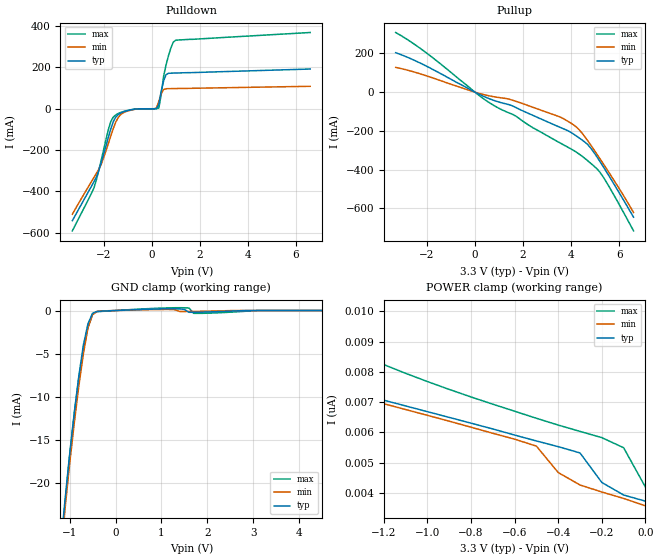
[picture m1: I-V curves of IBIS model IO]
|   TEXAS INSTRUMENTS INCORPORATED
|   Standard Linear and Logic
|   IBIS Model of SN74LVTH646
|   3.3V Octal Bus Transceiver Register (3-state)
|   24-pin DB, DGV, DW, or PW Package
[IBIS Ver]   2.1
[File Name]   lvth646.ibs
[File Rev]   1.0
[Date]   10/09/97
[Source]   File originated at Texas Instruments, Inc.
[Notes]   The following is an IBIS list for the LVTH646.
|   - This file may be incomplete or may not be fully compliant
|   with the IBIS specification. It will be replaced with a
|   version that is IBIS Revision 3.2 compliant and is complete
|   and accurate.  Please email all questions and comments to
|   sllibis@ti.com.
|   - All test data contained in this file are derived from
|   hspice(tm) simulations.
|   - File created by David Yaeger, SLL applications.
[Disclaimer]
* Property of Texas Instruments Incorporated.  Unauthorized *
* reproduction and/or distribution is strictly prohibited. *
* This product is protected under copyright law. *
* Created 1997, (C) Copyright 1997, Texas Instruments Inc., *
* All Rights Reserved *
* UNLESS THERE IS A SIGNED, WRITTEN AGREEMENT TO THE *
* CONTRARY, TEXAS INSTRUMENTS ("TI") IS PROVIDING THE IBIS *
* MODELS "AS IS" AND WITHOUT ANY WARRANTY, EXPRESSED OR *
* IMPLIED.  TI assumes no liability for: *
* 1) the accuracy of the IBIS models provided to your *
* company; *
* 2) the proper functioning of these IBIS models in your *
* design or for any resulting applications; or *
* 3) infringement of patents, copyrights or intellectual *
* property rights resulting from your use of these *
* IBIS models. *
* TI provides IBIS Models as a service to our customers. *
* You and your company shall not distribute, sell or give *
* these models to anyone else without prior written *
* permission from TI. *
* TI reserves the right to make changes to our products or *
* to discontinue any semiconductor product or service *
* without notice, and advises our customers to obtain the *
* latest version of relevant information to verify, before *
* placing orders, that the information being relied on is *
* current. *
* Please be aware that your receipt and use of the IBIS *
* information provided shall serve as acceptance of these *
* terms and conditions.  If you do not accept these terms, *
* you should return or destroy the IBIS models and any *
* other accompanying information immediately. *
[Component]   LVTH646_DB
[Manufacturer]  Texas Instruments, Inc.
[Package]
|   typ   min   max
R_pkg   0.045   0.04   0.049
L_pkg   3.668nH   3.226nH   4.415nH
C_pkg   0.416pF   0.349pF   0.507pF
[Pin]   signal_name   model_name   R_pin   L_pin   C_pin
1   CLKAB   NC   0.042   4.299nH   0.503pF
2   SAB   NC   0.04   3.96nH   0.499pF
3   DIR   NC   0.042   3.775nH   0.417pF
4   A1   IO   0.047   3.487nH   0.369pF
5   A2   IO   0.046   3.347nH   0.352pF
6   A3   IO   0.049   3.352nH   0.371pF
7   A4   IO   0.046   3.226nH   0.363pF
8   A5   IO   0.047   3.289nH   0.349pF
9   A6   IO   0.047   3.347nH   0.361pF
10   A7   IO   0.041   3.576nH   0.409pF
11   A8   IO   0.041   3.995nH   0.503pF
12   GND   GND   0.045   4.415nH   0.507pF
13   B8   IO   0.043   4.337nH   0.506pF
14   B7   IO   0.042   4.003nH   0.504pF
15   B6   IO   0.041   3.686nH   0.41pF
16   B5   IO   0.048   3.355nH   0.349pF
17   B4   IO   0.047   3.301nH   0.353pF
18   B3   IO   0.048   3.268nH   0.366pF
19   B2   IO   0.048   3.269nH   0.366pF
20   B1   IO   0.047   3.314nH   0.349pF
21   OE_BAR   NC   0.048   3.399nH   0.355pF
22   SBA   NC   0.041   3.688nH   0.412pF
23   CLKBA   NC   0.042   4.003nH   0.504pF
24   VCC   POWER   0.043   4.347nH   0.505pF
[Component]   LVTH646_DGV
[Manufacturer]  Texas Instruments, Inc.
[Package]
|   typ   min   max
R_pkg   0.043   0.039   0.047
L_pkg   2.601nH   2.312nH   3.626nH
C_pkg   0.358pF   0.277pF   0.595pF
[Pin]   signal_name   model_name   R_pin   L_pin   C_pin
1   CLKAB   NC   0.043   3.625nH   0.595pF
2   SAB   NC   0.04   2.656nH   0.402pF
3   DIR   NC   0.039   2.338nH   0.308pF
4   A1   IO   0.046   2.354nH   0.277pF
5   A2   IO   0.045   2.312nH   0.285pF
6   A3   IO   0.047   2.318nH   0.282pF
7   A4   IO   0.047   2.318nH   0.282pF
8   A5   IO   0.045   2.312nH   0.285pF
9   A6   IO   0.046   2.353nH   0.278pF
10   A7   IO   0.039   2.338nH   0.308pF
11   A8   IO   0.041   2.66nH   0.402pF
12   GND   GND   0.043   3.625nH   0.595pF
13   B8   IO   0.044   3.626nH   0.594pF
14   B7   IO   0.04   2.658nH   0.402pF
15   B6   IO   0.039   2.343nH   0.311pF
16   B5   IO   0.046   2.353nH   0.278pF
17   B4   IO   0.045   2.312nH   0.285pF
18   B3   IO   0.047   2.319nH   0.282pF
19   B2   IO   0.047   2.319nH   0.282pF
20   B1   IO   0.045   2.312nH   0.285pF
21   OE_BAR   NC   0.046   2.353nH   0.278pF
22   SBA   NC   0.039   2.337nH   0.308pF
23   CLKBA   NC   0.04   2.658nH   0.402pF
24   VCC   POWER   0.044   3.626nH   0.595pF
[Component]   LVTH646_DW
[Manufacturer]  Texas Instruments, Inc.
[Package]
|   typ   min   max
R_pkg   0.037   0.03   0.047
L_pkg   5.146nH   3.993nH   6.885nH
C_pkg   0.758pF   0.512pF   1.067pF
[Pin]   signal_name   model_name   R_pin   L_pin   C_pin
1   CLKAB   NC   0.039   6.885nH   1.067pF
2   SAB   NC   0.042   5.95nH   0.958pF
3   DIR   NC   0.047   5.317nH   0.791pF
4   A1   IO   0.031   4.651nH   0.611pF
5   A2   IO   0.03   3.993nH   0.512pF
6   A3   IO   0.03   4.083nH   0.611pF
7   A4   IO   0.03   4.083nH   0.611pF
8   A5   IO   0.03   3.993nH   0.512pF
9   A6   IO   0.031   4.652nH   0.611pF
10   A7   IO   0.047   5.317nH   0.791pF
11   A8   IO   0.042   5.95nH   0.959pF
12   GND   GND   0.039   6.885nH   1.067pF
13   B8   IO   0.039   6.885nH   1.067pF
14   B7   IO   0.042   5.95nH   0.959pF
15   B6   IO   0.047   5.317nH   0.791pF
16   B5   IO   0.031   4.652nH   0.611pF
17   B4   IO   0.03   3.993nH   0.512pF
18   B3   IO   0.03   4.083nH   0.61pF
19   B2   IO   0.03   4.083nH   0.61pF
20   B1   IO   0.03   3.993nH   0.512pF
21   OE_BAR   NC   0.031   4.651nH   0.611pF
22   SBA   NC   0.047   5.317nH   0.791pF
23   CLKBA   NC   0.042   5.95nH   0.958pF
24   VCC   POWER   0.039   6.885nH   1.067pF
[Component]   LVTH646_PW
[Manufacturer]  Texas Instruments, Inc.
[Package]
|   typ   min   max
R_pkg   0.039   0.03   0.046
L_pkg   2.685nH   2.367nH   3.177nH
C_pkg   0.32pF   0.252pF   0.434pF
[Pin]   signal_name   model_name   R_pin   L_pin   C_pin
1   CLKAB   NC   0.037   3.153nH   0.434pF
2   SAB   NC   0.034   2.629nH   0.341pF
3   DIR   NC   0.032   2.86nH   0.347pF
4   A1   IO   0.042   2.741nH   0.29pF
5   A2   IO   0.046   2.6nH   0.262pF
6   A3   IO   0.043   2.414nH   0.266pF
7   A4   IO   0.042   2.367nH   0.262pF
8   A5   IO   0.044   2.461nH   0.252pF
9   A6   IO   0.042   2.543nH   0.274pF
10   A7   IO   0.03   2.616nH   0.332pF
11   A8   IO   0.037   2.67nH   0.346pF
12   GND   GND   0.039   3.177nH   0.433pF
13   B8   IO   0.037   3.111nH   0.431pF
14   B7   IO   0.037   2.656nH   0.345pF
15   B6   IO   0.031   2.739nH   0.34pF
16   B5   IO   0.042   2.649nH   0.282pF
17   B4   IO   0.046   2.532nH   0.257pF
18   B3   IO   0.044   2.425nH   0.266pF
19   B2   IO   0.044   2.425nH   0.266pF
20   B1   IO   0.046   2.532nH   0.257pF
21   OE_BAR   NC   0.042   2.648nH   0.282pF
22   SBA   NC   0.031   2.738nH   0.339pF
23   CLKBA   NC   0.036   2.653nH   0.344pF
24   VCC   POWER   0.037   3.11nH   0.431pF
| Models and submodels in the file (1): IO (I/O)
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|   Model LVTH646_IO
[Model]   IO
Model_type   I/O
Polarity   Inverting
Enable   Active-Low
Vinl = 0.8V
Vinh = 2.0V
|   typ   min   max
C_comp   9pF   NA   NA
[Temperature Range]   50   0   100
[Voltage range]   3.3   3.0   3.6
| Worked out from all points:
|   slope of the pulldown table from 0 to 0.495 V, typ, clamps not added: 3.73 ohm
|   slope of the pullup table from 0 to 0.495 V, typ, clamps not added: 17.2 ohm
|   GND clamp passes 1 mA (typ) near -0.56 V on its own axis
[Pullup]   | Vtable = Vcc - Voutput
|   Voltage   I(typ)   I(min)   I(max)
-3.3V     203.6mA    127.8mA    307.8mA
-2V       132.9mA    83.47mA    200.5mA
500mV     -28.97mA   -16.47mA   -46.28mA
1.6V      -72.91mA   -43.01mA   -116.4mA
2.3V      -113.5mA   -72.99mA   -175.2mA
3.5V      -179.1mA   -126.1mA   -259mA
3.9V      -201.2mA   -152.7mA   -286.3mA
4.3V      -232.8mA   -189mA     -316.3mA
4.7V      -271.4mA   -251.8mA   -354.6mA
5.2V      -357.3mA   -342.7mA   -412.8mA
5.7V      -456.7mA   -438.2mA   -512.8mA
6.6V      -644.8mA   -620.7mA   -715.4mA
[Pulldown]
|   Voltage   I(typ)   I(min)   I(max)
-3.3V     -541.1mA   -510mA     -590.2mA
-2.4V     -352.7mA   -331.9mA   -382.4mA
-2.1V     -260.9mA   -270.2mA   -249.8mA
-1.8V     -138mA     -167.8mA   -100.2mA
-1.5V     -41.84mA   -66.63mA   -30.62mA
-1.2V     -16.44mA   -21.07mA   -14.61mA
200mV     117.8uA    3.002mA    -393.7uA
300mV     19.97mA    35.86mA    3.638mA
500mV     134.6mA    92.85mA    157.4mA
600mV     164.2mA    96.34mA    211.3mA
900mV     171.9mA    97.14mA    321.3mA
6.6V      191.6mA    108.1mA    368mA
[POWER_Clamp]   | Vtable = Vcc - Voutput
|   Voltage   I(typ)   I(min)   I(max)
-3.3V     11.05nA    10.98nA    33.46nA
-2.8V     10.1nA     10.02nA    20.04nA
-2.7V     9.915nA    9.827nA    18.39nA
-1.7V     8.016nA    7.91nA     10.03nA
-1.4V     7.447nA    7.334nA    8.877nA
-1.2V     7.067nA    6.951nA    8.244nA
-500mV    5.719nA    5.549nA    6.469nA
-400mV    5.532nA    4.676nA    6.245nA
-300mV    5.324nA    4.264nA    6.035nA
-200mV    4.348nA    4.032nA    5.83nA
-100mV    3.933nA    3.82nA     5.496nA
0V        3.73nA     3.575nA    4.195nA
[GND_Clamp]
|   Voltage   I(typ)   I(min)   I(max)
-3.3V     -592.4mA   -565mA     -637.9mA
-1.2V     -27.61mA   -29.28mA   -28.29mA
-1.1V     -21.96mA   -23mA      -22.3mA
-900mV    -11.92mA   -13.08mA   -12.07mA
-800mV    -7.594mA   -8.784mA   -7.919mA
-700mV    -3.984mA   -5.016mA   -4.574mA
-600mV    -1.527mA   -2.003mA   -1.963mA
-500mV    -312.1uA   -481.1uA   -411.8uA
1.3V      200.3uA    84.62uA    322.1uA
1.6V      -205.7uA   -110.8uA   288uA
1.7V      -203.5uA   -104.1uA   -327.6uA
6.6V      11.05nA    11.55nA    24.19nA
[Ramp]
| variable   typ   min   max
dV/dt_r   1.4656E+00/2.9694E-10  1.1366E+00/6.8901E-10  1.7471E+00/1.8592E-10
dV/dt_f   1.7801E+00/7.7452E-10  1.6010E+00/1.2118E-09  1.9610E+00/5.1776E-10
